| TEXAS INSTRUMENTS INCORPORATED
| Standard Linear and Logic Group
| IBIS Model of SN74CBTLV16800
| LOW-VOLTAGE 20-BIT FET BUS SWITCH WITH PRECHARGED OUTPUTS
| This file contains package information for the following:
|  TSSOP 48-pin (DGG) package as [Component] CBTLV16800_DGG
|  TVSOP 48-pin (DGV) package as [Component] CBTLV16800_DGV
|  SSOP 48-pin (DL) package as [Component] CBTLV16800_DL
| This device can be powered at the following Vccs:
|  2.5 volt Vcc
|  3.3 volt Vcc
| This file provides unique models under the [Model Selector] for each Vcc.
| For operation at a specific Vcc, select the appropriate model after each
| [Model Selector] keyword.
[IBIS Ver]   3.2
[Comment char]  |_char
[File Name]   sn74cbtlv16800.ibs
[File Rev]   1.1 | c_die
[Date]   August 2, 2002
[Source]   Data created from TI-SPICE simulations at TI-SLL.
[Notes]   The following is an IBIS list for the CBTLV16800.
   Please contact sllibis@ti.com with questions and
   comments concerning SLL IBIS models.
   - As there is no power clamp diode in the Input and Output
   Models, we removed the Pwr Clamp table data from those
   Models.
   - Non-monotonic data due to FET characteristics.
[Disclaimer] Property of Texas Instruments Incorporated.  Unauthorized
   reproduction and/or distribution is strictly prohibited.
   This product is protected under copyright law.
   Created  2002, (C) Copyright  2002, Texas Instruments
   Incorporated, All Rights Reserved
   UNLESS THERE IS A SIGNED, WRITTEN AGREEMENT TO THE
   CONTRARY, TEXAS INSTRUMENTS (TI) IS PROVIDING THE IBIS
   MODELS  AND WITHOUT ANY WARRANTY, EXPRESSED OR
   IMPLIED.  TI assumes no liability for:
   1) the accuracy of the IBIS models provided to your
   company;
   2) the proper functioning of these IBIS Models in your
   design or for any resulting applications; or
   3) infringement of patents, copyrights or intellectual
   property rights resulting from your use of these IBIS
   models.
   TI provides IBIS Models as a service to our customers.
   You and your company shall not distribute, sell or give
   these models to anyone else without prior written
   permission from TI.
   TI reserves the right to make changes to our products or
   to discontinue any semiconductor product or service
   without notice, and advises our customers to obtain the
   latest version of relevant information to verify, before
   placing orders, that the information being relied on is
   current.
   Please be aware that your receipt and use of the IBIS
   information provided shall serve as acceptance of these
   terms and conditions.  If you do not accept these terms,
   you should return or destroy the IBIS models and any
   other accompanying information immediately.
| Component CBTLV16800_DGG 48-pin TSSOP
[Component]   CBTLV16800_DGG
[Manufacturer]   Texas Instruments, Inc.
[Package]
|   typ   min   max
R_pkg   4.400e-02   3.800e-02   5.100e-02
L_pkg   3.019e-09   2.486e-09   4.099e-09
C_pkg   5.070e-13   3.340e-13   8.090e-13
[Pin]   signal_name   model_name   R_pin   L_pin   C_pin
1   BIASV   POWER   4.100e-02   4.017e-09   7.590e-13
2   1A1   CBTLV16800_IO   4.200e-02   3.737e-09   7.920e-13
3   1A2   CBTLV16800_IO   4.200e-02   3.480e-09   6.610e-13
4   1A3   CBTLV16800_IO   3.800e-02   3.131e-09   5.750e-13
5   1A4   CBTLV16800_IO   4.700e-02   3.122e-09   5.660e-13
6   1A5   CBTLV16800_IO   4.300e-02   2.948e-09   5.040e-13
7   1A6   CBTLV16800_IO   4.500e-02   2.845e-09   3.970e-13
8   GND   GND   4.900e-02   2.835e-09   3.940e-13
9   1A7   CBTLV16800_IO   4.800e-02   2.715e-09   3.780e-13
10   1A8   CBTLV16800_IO   5.000e-02   2.664e-09   3.630e-13
11   1A9   CBTLV16800_IO   5.000e-02   2.585e-09   3.480e-13
12   1A10   CBTLV16800_IO   4.900e-02   2.550e-09   3.370e-13
13   2A1   CBTLV16800_IO   4.900e-02   2.541e-09   3.360e-13
14   2A2   CBTLV16800_IO   5.000e-02   2.574e-09   3.480e-13
15   VCC   POWER   4.900e-02   2.618e-09   3.590e-13
16   2A3   CBTLV16800_IO   4.600e-02   2.671e-09   3.750e-13
17   GND   GND   4.500e-02   2.754e-09   3.890e-13
18   2A4   CBTLV16800_IO   4.400e-02   2.823e-09   4.500e-13
19   2A5   CBTLV16800_IO   4.200e-02   2.968e-09   5.030e-13
20   2A6   CBTLV16800_IO   5.100e-02   3.108e-09   5.350e-13
21   2A7   CBTLV16800_IO   4.200e-02   3.175e-09   5.870e-13
22   2A8   CBTLV16800_IO   4.100e-02   3.449e-09   6.780e-13
23   2A9   CBTLV16800_IO   4.400e-02   3.766e-09   8.040e-13
24   2A10   CBTLV16800_IO   4.300e-02   4.065e-09   7.610e-13
25   2B10   CBTLV16800_IO   4.100e-02   3.994e-09   7.570e-13
26   2B9   CBTLV16800_IO   3.900e-02   3.649e-09   7.890e-13
27   2B8   CBTLV16800_IO   3.800e-02   3.362e-09   6.600e-13
28   2B7   CBTLV16800_IO   3.800e-02   3.082e-09   5.740e-13
29   2B6   CBTLV16800_IO   4.400e-02   2.990e-09   5.220e-13
30   2B5   CBTLV16800_IO   4.100e-02   2.917e-09   4.950e-13
31   2B4   CBTLV16800_IO   4.300e-02   2.820e-09   4.480e-13
32   GND   GND   4.300e-02   2.699e-09   3.850e-13
33   2B3   CBTLV16800_IO   4.500e-02   2.628e-09   3.720e-13
34   2B2   CBTLV16800_IO   4.600e-02   2.556e-09   3.560e-13
35   2B1   CBTLV16800_IO   4.600e-02   2.495e-09   3.440e-13
36   1B10   CBTLV16800_IO   4.700e-02   2.487e-09   3.340e-13
37   1B9   CBTLV16800_IO   4.700e-02   2.490e-09   3.350e-13
38   1B8   CBTLV16800_IO   4.600e-02   2.486e-09   3.430e-13
39   1B7   CBTLV16800_IO   4.500e-02   2.566e-09   3.560e-13
40   1B6   CBTLV16800_IO   4.400e-02   2.639e-09   3.740e-13
41   GND   GND   4.300e-02   2.701e-09   3.860e-13
42   1B5   CBTLV16800_IO   4.300e-02   2.817e-09   4.500e-13
43   1B4   CBTLV16800_IO   4.100e-02   2.935e-09   5.010e-13
44   1B3   CBTLV16800_IO   4.700e-02   3.035e-09   5.290e-13
45   1B2   CBTLV16800_IO   4.300e-02   3.171e-09   5.890e-13
46   1B1   CBTLV16800_IO   4.000e-02   3.415e-09   6.820e-13
47   2OE   CBTLV16800_NOE   4.300e-02   3.741e-09   8.090e-13
48   1OE   CBTLV16800_NOE   4.400e-02   4.099e-09   7.640e-13
| Component CBTLV16800_DGV 48-pin TVSOP
[Component]   CBTLV16800_DGV
[Manufacturer]   Texas Instruments, Inc.
[Package]
|   typ   min   max
R_pkg   7.000e-02   4.900e-02   8.500e-02
L_pkg   3.013e-09   2.743e-09   3.408e-09
C_pkg   3.710e-13   2.940e-13   5.110e-13
[Pin]   signal_name   model_name   R_pin   L_pin   C_pin
1   BIASV   POWER   4.900e-02   3.393e-09   4.970e-13
2   1A1   CBTLV16800_IO   6.000e-02   3.250e-09   5.020e-13
3   1A2   CBTLV16800_IO   7.700e-02   3.310e-09   4.510e-13
4   1A3   CBTLV16800_IO   8.500e-02   3.299e-09   4.040e-13
5   1A4   CBTLV16800_IO   8.300e-02   3.136e-09   3.600e-13
6   1A5   CBTLV16800_IO   7.700e-02   3.019e-09   3.630e-13
7   1A6   CBTLV16800_IO   6.500e-02   2.882e-09   3.490e-13
8   GND   GND   6.600e-02   2.829e-09   3.140e-13
9   1A7   CBTLV16800_IO   6.700e-02   2.796e-09   3.140e-13
10   1A8   CBTLV16800_IO   6.900e-02   2.754e-09   3.080e-13
11   1A9   CBTLV16800_IO   7.000e-02   2.753e-09   3.010e-13
12   1A10   CBTLV16800_IO   7.100e-02   2.745e-09   2.940e-13
13   2A1   CBTLV16800_IO   7.000e-02   2.744e-09   2.940e-13
14   2A2   CBTLV16800_IO   7.000e-02   2.754e-09   3.010e-13
15   VCC   POWER   6.900e-02   2.754e-09   3.080e-13
16   2A3   CBTLV16800_IO   6.700e-02   2.796e-09   3.140e-13
17   GND   GND   6.600e-02   2.829e-09   3.140e-13
18   2A4   CBTLV16800_IO   6.500e-02   2.883e-09   3.500e-13
19   2A5   CBTLV16800_IO   7.500e-02   3.014e-09   3.630e-13
20   2A6   CBTLV16800_IO   8.000e-02   3.128e-09   3.580e-13
21   2A7   CBTLV16800_IO   8.400e-02   3.295e-09   4.030e-13
22   2A8   CBTLV16800_IO   7.800e-02   3.311e-09   4.520e-13
23   2A9   CBTLV16800_IO   6.200e-02   3.259e-09   5.010e-13
24   2A10   CBTLV16800_IO   5.200e-02   3.404e-09   4.960e-13
25   2B10   CBTLV16800_IO   5.300e-02   3.397e-09   5.050e-13
26   2B9   CBTLV16800_IO   6.200e-02   3.249e-09   5.110e-13
27   2B8   CBTLV16800_IO   7.700e-02   3.308e-09   4.530e-13
28   2B7   CBTLV16800_IO   8.200e-02   3.289e-09   4.030e-13
29   2B6   CBTLV16800_IO   7.800e-02   3.121e-09   3.590e-13
30   2B5   CBTLV16800_IO   7.400e-02   3.010e-09   3.630e-13
31   2B4   CBTLV16800_IO   6.500e-02   2.883e-09   3.490e-13
32   GND   GND   6.700e-02   2.829e-09   3.140e-13
33   2B3   CBTLV16800_IO   6.700e-02   2.795e-09   3.140e-13
34   2B2   CBTLV16800_IO   6.900e-02   2.753e-09   3.070e-13
35   2B1   CBTLV16800_IO   7.000e-02   2.753e-09   3.010e-13
36   1B10   CBTLV16800_IO   7.000e-02   2.743e-09   2.940e-13
37   1B9   CBTLV16800_IO   7.000e-02   2.743e-09   2.940e-13
38   1B8   CBTLV16800_IO   7.000e-02   2.753e-09   3.010e-13
39   1B7   CBTLV16800_IO   6.900e-02   2.754e-09   3.070e-13
40   1B6   CBTLV16800_IO   6.800e-02   2.797e-09   3.140e-13
41   GND   GND   6.700e-02   2.830e-09   3.140e-13
42   1B5   CBTLV16800_IO   6.400e-02   2.880e-09   3.490e-13
43   1B4   CBTLV16800_IO   7.200e-02   3.004e-09   3.620e-13
44   1B3   CBTLV16800_IO   7.800e-02   3.121e-09   3.590e-13
45   1B2   CBTLV16800_IO   8.400e-02   3.296e-09   4.030e-13
46   1B1   CBTLV16800_IO   7.700e-02   3.308e-09   4.510e-13
47   2OE   CBTLV16800_NOE   6.200e-02   3.258e-09   4.990e-13
48   1OE   CBTLV16800_NOE   5.300e-02   3.408e-09   4.940e-13
| Component CBTLV16800_DL 48-pin SSOP
[Component]   CBTLV16800_DL
[Manufacturer]   Texas Instruments, Inc.
[Package]
|   typ   min   max
R_pkg   4.800e-02   3.800e-02   5.300e-02
L_pkg   6.046e-09   5.084e-09   7.968e-09
C_pkg   8.130e-13   5.690e-13   1.157e-12
[Pin]   signal_name   model_name   R_pin   L_pin   C_pin
1   BIASV   POWER   4.600e-02   7.968e-09   1.017e-12
2   1A1   CBTLV16800_IO   4.400e-02   7.299e-09   1.157e-12
3   1A2   CBTLV16800_IO   4.300e-02   6.765e-09   1.058e-12
4   1A3   CBTLV16800_IO   4.100e-02   6.269e-09   9.330e-13
5   1A4   CBTLV16800_IO   3.800e-02   5.856e-09   8.290e-13
6   1A5   CBTLV16800_IO   4.600e-02   5.802e-09   7.900e-13
7   1A6   CBTLV16800_IO   5.000e-02   5.656e-09   7.380e-13
8   GND   GND   5.300e-02   5.500e-09   6.430e-13
9   1A7   CBTLV16800_IO   5.200e-02   5.304e-09   6.060e-13
10   1A8   CBTLV16800_IO   5.300e-02   5.189e-09   5.830e-13
11   1A9   CBTLV16800_IO   5.100e-02   5.084e-09   5.690e-13
12   1A10   CBTLV16800_IO   5.300e-02   5.862e-09   8.330e-13
13   2A1   CBTLV16800_IO   5.300e-02   5.862e-09   8.330e-13
14   2A2   CBTLV16800_IO   5.100e-02   5.084e-09   5.690e-13
15   VCC   POWER   5.300e-02   5.189e-09   5.830e-13
16   2A3   CBTLV16800_IO   5.200e-02   5.304e-09   6.060e-13
17   GND   GND   5.300e-02   5.500e-09   6.430e-13
18   2A4   CBTLV16800_IO   5.000e-02   5.656e-09   7.380e-13
19   2A5   CBTLV16800_IO   4.600e-02   5.802e-09   7.900e-13
20   2A6   CBTLV16800_IO   3.800e-02   5.856e-09   8.290e-13
21   2A7   CBTLV16800_IO   4.100e-02   6.269e-09   9.330e-13
22   2A8   CBTLV16800_IO   4.300e-02   6.765e-09   1.058e-12
23   2A9   CBTLV16800_IO   4.400e-02   7.299e-09   1.157e-12
24   2A10   CBTLV16800_IO   4.600e-02   7.968e-09   1.017e-12
25   2B10   CBTLV16800_IO   4.600e-02   7.968e-09   1.017e-12
26   2B9   CBTLV16800_IO   4.400e-02   7.299e-09   1.157e-12
27   2B8   CBTLV16800_IO   4.300e-02   6.765e-09   1.058e-12
28   2B7   CBTLV16800_IO   4.100e-02   6.269e-09   9.330e-13
29   2B6   CBTLV16800_IO   3.800e-02   5.856e-09   8.290e-13
30   2B5   CBTLV16800_IO   4.600e-02   5.802e-09   7.900e-13
31   2B4   CBTLV16800_IO   5.000e-02   5.656e-09   7.380e-13
32   GND   GND   5.300e-02   5.500e-09   6.430e-13
33   2B3   CBTLV16800_IO   5.200e-02   5.304e-09   6.060e-13
34   2B2   CBTLV16800_IO   5.300e-02   5.189e-09   5.830e-13
35   2B1   CBTLV16800_IO   5.100e-02   5.084e-09   5.690e-13
36   1B10   CBTLV16800_IO   5.300e-02   5.862e-09   8.330e-13
37   1B9   CBTLV16800_IO   5.300e-02   5.862e-09   8.330e-13
38   1B8   CBTLV16800_IO   5.100e-02   5.084e-09   5.690e-13
39   1B7   CBTLV16800_IO   5.300e-02   5.189e-09   5.830e-13
40   1B6   CBTLV16800_IO   5.200e-02   5.304e-09   6.060e-13
41   GND   GND   5.300e-02   5.500e-09   6.430e-13
42   1B5   CBTLV16800_IO   5.000e-02   5.656e-09   7.380e-13
43   1B4   CBTLV16800_IO   4.600e-02   5.802e-09   7.900e-13
44   1B3   CBTLV16800_IO   3.800e-02   5.856e-09   8.290e-13
45   1B2   CBTLV16800_IO   4.100e-02   6.269e-09   9.330e-13
46   1B1   CBTLV16800_IO   4.300e-02   6.765e-09   1.058e-12
47   2OE   CBTLV16800_NOE   4.400e-02   7.299e-09   1.157e-12
48   1OE   CBTLV16800_NOE   4.600e-02   7.967e-09   1.017e-12
[Series Switch Groups]
| Function Group States
On  1 /   | 1A1-1A10->1B1-1B10 1NOE, LOW
On  2 /   | 2A1-2A10->2B1-2B10 2NOE, LOW
On  1 2 /   | 1NOE, LOW, 2NOE, LOW
[Series Pin Mapping]   pin_2   model_name   function_table_group
2   46   CBTLV16800_IO_25_S   1
| 2   46   CBTLV16800_IO_33_S   1
3   45   CBTLV16800_IO_25_S   1
| 3   45   CBTLV16800_IO_33_S   1
4   44   CBTLV16800_IO_25_S   1
| 4   44   CBTLV16800_IO_33_S   1
5   43   CBTLV16800_IO_25_S   1
| 5   43   CBTLV16800_IO_33_S   1
6   42   CBTLV16800_IO_25_S   1
| 6   42   CBTLV16800_IO_33_S   1
7   40   CBTLV16800_IO_25_S   1
| 7   40   CBTLV16800_IO_33_S   1
9   39   CBTLV16800_IO_25_S   1
| 9   39   CBTLV16800_IO_33_S   1
10   38   CBTLV16800_IO_25_S   1
| 10   38   CBTLV16800_IO_33_S   1
11   37   CBTLV16800_IO_25_S   1
| 11   37   CBTLV16800_IO_33_S   1
12   36   CBTLV16800_IO_25_S   1
| 12   36   CBTLV16800_IO_33_S   1
13   35   CBTLV16800_IO_25_S   2
| 13   35   CBTLV16800_IO_33_S   2
14   34   CBTLV16800_IO_25_S   2
| 14   34   CBTLV16800_IO_33_S   2
16   33   CBTLV16800_IO_25_S   2
| 16   33   CBTLV16800_IO_33_S   2
18   31   CBTLV16800_IO_25_S   2
| 18   31   CBTLV16800_IO_33_S   2
19   30   CBTLV16800_IO_25_S   2
| 19   30   CBTLV16800_IO_33_S   2
20   29   CBTLV16800_IO_25_S   2
| 20   29   CBTLV16800_IO_33_S   2
21   28   CBTLV16800_IO_25_S   2
| 21   28   CBTLV16800_IO_33_S   2
22   27   CBTLV16800_IO_25_S   2
| 22   27   CBTLV16800_IO_33_S   2
23   26   CBTLV16800_IO_25_S   2
| 23   26   CBTLV16800_IO_33_S   2
24   25   CBTLV16800_IO_25_S   2
| 24   25   CBTLV16800_IO_33_S   2
| Model CBTLV16800_NOE
[Model Selector]   CBTLV16800_NOE
CBTLV16800_NOE_25   2.5 volt Vcc
CBTLV16800_NOE_33   3.3 volt Vcc
| Model CBTLV16800_IO
[Model Selector]   CBTLV16800_IO
CBTLV16800_IO_25   2.5 volt Vcc
CBTLV16800_IO_33   3.3 volt Vcc
| Model CBTLV16800_IO_S
[Model Selector]   CBTLV16800_IO_S
CBTLV16800_IO_25_S   2.5 volt Vcc
CBTLV16800_IO_33_S   3.3 volt Vcc
[Model]   CBTLV16800_IO_25_S
Model_type  Series_switch
| variable   typ   min   max
C_comp   0   0   0
[Temperature Range]   40   100   -40
| Ambient temperature   25   85   -40
[Voltage range]   2.5   2.3   2.7
[On]
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[Off]
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[Model]   CBTLV16800_IO_33_S
Model_type  Series_switch
| variable   typ   min   max
C_comp   0   0   0
[Temperature Range]   40   100   -40
| Ambient temperature   25   85   -40
[Voltage range]   3.3   3   3.6
[On]
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[Off]
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| Models and submodels in the file (6): CBTLV16800_NOE_25 (Input), CBTLV16800_NOE_33 (Input), CBTLV16800_IO_25_S (Series_switch), CBTLV16800_IO_25 (Terminator), CBTLV16800_IO_33_S (Series_switch), CBTLV16800_IO_33 (Terminator)
